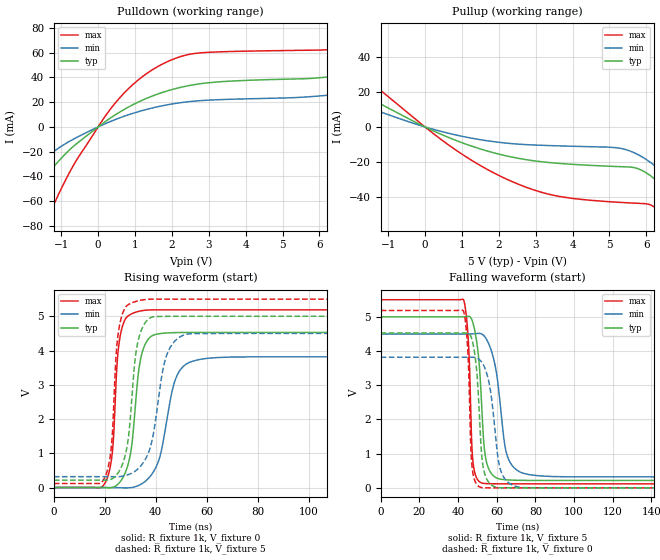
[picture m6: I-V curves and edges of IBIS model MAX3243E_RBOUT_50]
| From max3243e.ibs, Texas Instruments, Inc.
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[Model]   MAX3243E_RBOUT_50
Model_type  Output
Vref =   0
Rref =   3000
Cref =   150p
Vmeas =   1.5
| variable   typ   min   max
C_comp   4.44pF   3.21pF   7.17pF
| C_pullup   4.13pF   3.21pF   5.34pF
| C_pulldown   4.74pF   3.34pF   7.17pF
[Temperature Range]   40   100   -40
| Ambient temperature   25   85   -40
[Voltage range]   5   4.5   5.5
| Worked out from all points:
|   slope of the pulldown table from 0 to 0.75 V, typ, clamps not added: 50.5 ohm
|   slope of the pullup table from 0 to 0.75 V, typ, clamps not added: 108 ohm
|   rising waveform, R_fixture 1k, V_fixture 0: 20-80 % time 3.86ns typ, 6.23ns min, 2.51ns max; typ from 0 V to 4.53 V
|   falling waveform, R_fixture 1k, V_fixture 5: 20-80 % time 3.39ns typ, 5.64ns min, 1.99ns max; typ from 5 V to 0.216 V
|   rising waveform, R_fixture 1k, V_fixture 5: 20-80 % time 3.76ns typ, 5.71ns min, 2.57ns max; typ from 0.216 V to 5 V
|   falling waveform, R_fixture 1k, V_fixture 0: 20-80 % time 3.03ns typ, 4.9ns min, 1.84ns max; typ from 4.53 V to 0 V
[Pulldown]
| MAX3243E_RBOUT_50
|   Voltage   I(typ)   I(min)   I(max)
-5V       -225.3mA   -151.9mA   -353.7mA
-3.3V     -128.7mA   -83.23mA   -222mA
-2.39V    -82.12mA   -51.8mA    -149.7mA
-1.515V   -43.74mA   -27.04mA   -84.05mA
-625mV    -14.57mA   -9.2mA     -28.83mA
430mV     9.101mA    5.545mA    18.05mA
1.23V     22.01mA    13.5mA     41.26mA
2.17V     31.51mA    19.31mA    56.21mA
3V        35.72mA    21.67mA    60.29mA
6.635V    41.93mA    26.92mA    63.99mA
8.425V    52.64mA    35.07mA    78.79mA
10V       65.5mA     44.8mA     96.53mA
[Pullup]
| MAX3243E_RBOUT_50
|   Voltage   I(typ)   I(min)   I(max)
-5V       55.24mA    39.06mA    81.51mA
-3.28V    36.3mA     24.83mA    55.11mA
675mV     -6.314mA   -3.785mA   -10.8mA
2.74V     -18.63mA   -10.07mA   -34.31mA
3.88V     -21.12mA   -10.93mA   -40.34mA
5.68V     -23.19mA   -14.78mA   -43.37mA
6.125V    -27.97mA   -20.41mA   -44.5mA
6.415V    -33.4mA    -25.44mA   -49.55mA
6.69V     -40.02mA   -31.12mA   -57.74mA
7.205V    -55.75mA   -43.95mA   -79.43mA
7.7V      -74.32mA   -58.64mA   -105.9mA
10V       -188.4mA   -147.8mA   -262.8mA
[Ramp]
| MAX3243E_RBOUT_50
| variable   typ   min   max
dV/dt_r   2.72/3.87E-09   2.30/6.25E-09   3.12/2.52E-09
dV/dt_f   2.88/3.40E-09   2.52/5.67E-09   3.24/2.00E-09
R_load = 1k
[Rising Waveform]
| MAX3243E_RBOUT_50
R_fixture =   1k
C_fixture =   0
L_fixture =   0
V_fixture =   0
V_fixture_min = 0
V_fixture_max = 0
|   Time   V(typ)   V(min)   V(max)
0s        591.1pV    1.593nV    266.5pV
20.4ns    -3.882mV   25.46uV    173.6mV
23ns      -255.6uV   98.42uV    1.049V
26.1ns    175.8mV    -6.834mV   4.443V
30.2ns    1.028V     -3.255mV   5.057V
33.2ns    3.337V     58.55mV    5.141V
41.1ns    4.487V     772.3mV    5.187V
48.4ns    4.523V     3.276V     5.187V
56.7ns    4.528V     3.731V     5.187V
269.9ns   4.528V     3.818V     5.187V
[Falling Waveform]
| MAX3243E_RBOUT_50
R_fixture =   1k
C_fixture =   0
L_fixture =   0
V_fixture =   5
V_fixture_min = 4.5
V_fixture_max = 5.5
|   Time   V(typ)   V(min)   V(max)
0s        5V         4.5V       5.5V
42.8ns    5.001V     4.5V       5.502V
45.4ns    5.017V     4.5V       4.225V
47.7ns    4.822V     4.503V     767.2mV
52.2ns    2.434V     4.499V     142.4mV
53.8ns    1.051V     4.419V     128.3mV
56.4ns    491.1mV    4.139V     121.3mV
65ns      235.2mV    1.022V     117.4mV
73.6ns    219.4mV    427.6mV    117.2mV
269.9ns   216.3mV    317.4mV    117.2mV
[Rising Waveform]
| MAX3243E_RBOUT_50
R_fixture =   1k
C_fixture =   0
L_fixture =   0
V_fixture =   5
V_fixture_min = 4.5
V_fixture_max = 5.5
|   Time   V(typ)   V(min)   V(max)
0s        216.3mV    317.4mV    117.2mV
20.1ns    215.1mV    317.4mV    303.8mV
22.6ns    244.4mV    317.2mV    1.206V
25.7ns    481.8mV    318.5mV    4.692V
29.1ns    1.352V     374mV      5.333V
32.8ns    4.182V     529.5mV    5.446V
38.3ns    4.969V     1.286V     5.498V
44.3ns    4.997V     3.861V     5.5V
52ns      5V         4.473V     5.5V
269.9ns   5V         4.5V       5.5V
[Falling Waveform]
| MAX3243E_RBOUT_50
R_fixture =   1k
C_fixture =   0
L_fixture =   0
V_fixture =   0
V_fixture_min = 0
V_fixture_max = 0
|   Time   V(typ)   V(min)   V(max)
0s        4.528V     3.818V     5.187V
42.7ns    4.529V     3.818V     5.179V
45ns      4.523V     3.819V     4.048V
47.2ns    4.332V     3.819V     639.4mV
49.7ns    3.384V     3.797V     98.88mV
51.7ns    1.39V      3.712V     13.86mV
56.4ns    126.5mV    2.961V     822.4uV
61.8ns    4.221mV    556.1mV    218.9uV
69.8ns    815uV      44.79mV    91.75uV
269.9ns   1.775nV    2.361nV    287.9pV
